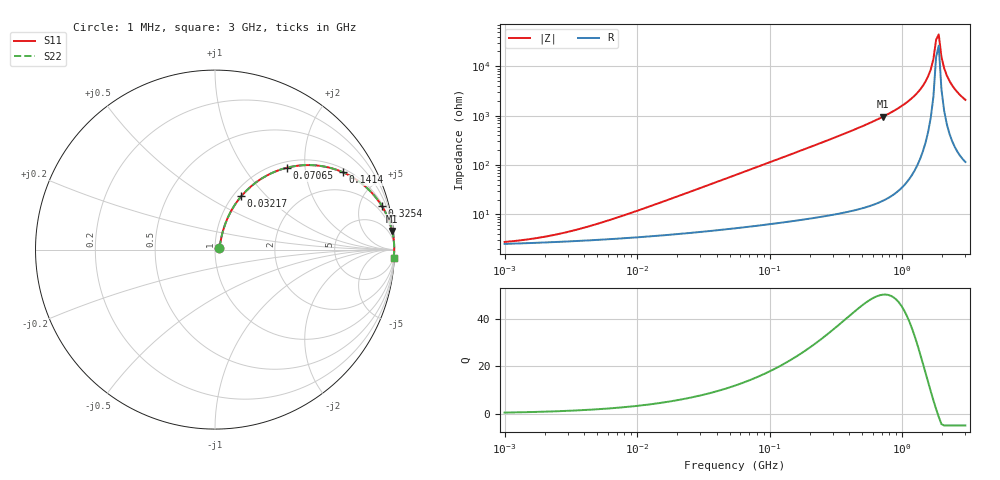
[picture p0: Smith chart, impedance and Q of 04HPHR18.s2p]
# MHz S MA R 50
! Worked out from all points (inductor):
!   174 points, 1 MHz to 3 GHz, reference 50 ohm
!   read as one part in series: L = 180 nH near 9.22 MHz
!   highest Q = 50.5 at 714.6 MHz (marker M1), where L = 211 nH
!   self-resonance near 1.803 GHz
!   S11 on the Smith chart (normalised r, x): 1 MHz: 1.05, +0.02; 32.17 MHz: 1.09, +0.73; 70.65 MHz: 1.11, +1.60; 141.4 MHz: 1.14, +3.22; 325.4 MHz: 1.20, +7.59; 3 GHz: 3, -42
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1  0.02694 23.5  0.9754 -0.6  0.9754 -0.6  0.02694 23.5
3.8271  0.05069 53.6  0.9708 -2.4  0.9708 -2.4  0.05069 53.6
14.6467  0.1616 68.3  0.9522 -9.1  0.9522 -9.1  0.1616 68.3
32.1679  0.3314 63.8  0.9038 -19.2  0.9038 -19.2  0.3314 63.8
56.0545  0.5181 54.2  0.8137 -31.1  0.8137 -31.1  0.5181 54.2
70.6488  0.6053 48.8  0.7546 -37.1  0.7546 -37.1  0.6053 48.8
141.446  0.8332 31.1  0.5173 -56.3  0.5173 -56.3  0.8332 31.1
214.526  0.9155 21.8  0.3721 -66.2  0.3721 -66.2  0.9155 21.8
325.365  0.9607 14.6  0.2529 -73.8  0.2529 -73.8  0.9607 14.6
714.584  0.9925 6.0  0.1045 -82.9  0.1045 -82.9  0.9925 6.0
821.013  0.9946 4.9  0.08607 -83.9  0.08607 -83.9  0.9946 4.9
1188.89  0.9978 2.5  0.04366 -85.9  0.04366 -85.9  0.9978 2.5
1498.43  0.9986 1.2  0.02041 -85.5  0.02041 -85.5  0.9986 1.2
1643.75  0.9987 0.7  0.0115 -83.3  0.0115 -83.3  0.9987 0.7
1721.61  0.9987 0.4  0.007119 -79.5  0.007119 -79.5  0.9987 0.4
1803.15  0.9987 0.1  0.002897 -63.4  0.002897 -63.4  0.9987 0.1
1888.56  0.9987 -0.1  0.002259 53.4  0.002259 53.4  0.9987 -0.1
1978.02  0.9986 -0.4  0.006385 76.9  0.006385 76.9  0.9986 -0.4
2071.71  0.9985 -0.6  0.01075 81.4  0.01075 81.4  0.9985 -0.6
2169.84  0.9983 -0.9  0.01518 83.2  0.01518 83.2  0.9983 -0.9
2493.02  0.9977 -1.6  0.02871 84.5  0.02871 84.5  0.9977 -1.6
3000  0.9962 -2.7  0.04763 84.1  0.04763 84.1  0.9962 -2.7
